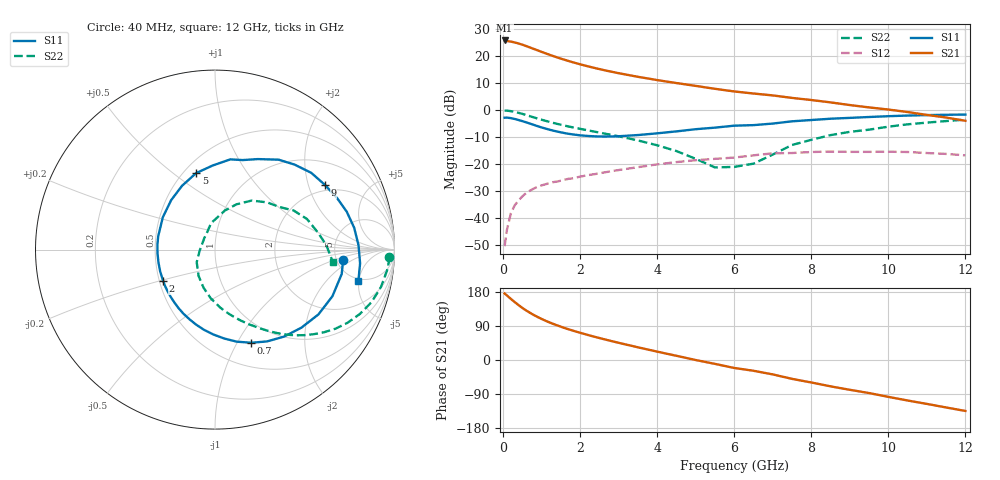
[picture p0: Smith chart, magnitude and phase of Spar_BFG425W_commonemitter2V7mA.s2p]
! Filename: 27bfg425.001
! BFG425W Field C1
! V1=8.380E-001V,V2=2.000E+000V, I1=9.357E-005A, I2=6.990E-003A
# GHz  S  MA  R 50
!  S11  S21  S12  S22
!Freq(GHz)  Mag  Ang  Mag  Ang  Mag  Ang  Mag  Ang
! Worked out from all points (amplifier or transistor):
!   44 points, 40 MHz to 12 GHz, reference 50 ohm
!   highest |S21| = 25.7 dB at 40 MHz (marker M1)
!   |S21| within 3 dB of that: start of sweep to 772.9 MHz
!   unconditionally stable (mu >= 1): 2.179 GHz to end of sweep
!   at 700 MHz: K = 0.42, MSG = 26.5 dB, |S12| = -29.9 dB
!   at 2.4 GHz: K = 1.06, MAG = 18.1 dB, |S12| = -23.7 dB
!   at 12 GHz: K = 1.43, MAG = 2.5 dB, |S12| = -16.8 dB
!   S11 on the Smith chart (normalised r, x): 40 MHz: 5.73, -1.33; 700 MHz: 0.76, -1.15; 2 GHz: 0.52, -0.21; 5 GHz: 0.58, +0.61; 9 GHz: 1.77, +2.58; 12 GHz: 4.61, -4.92
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0.04  0.716 -4.5  19.28 175.5  0.003 83.5  0.973 -2.4
0.2  0.704 -21.7  18.38 161.3  0.012 77.7  0.948 -12.7
0.3  0.68 -32.1  17.73 153.1  0.017 72.7  0.92 -18.6
0.4  0.649 -42.0  16.95 145.1  0.021 67.8  0.883 -24.0
0.5  0.619 -51.5  16.11 137.4  0.025 63.5  0.844 -28.8
0.6  0.588 -60.5  15.18 130.6  0.029 59.6  0.804 -33.2
0.7  0.557 -68.7  14.27 124.5  0.032 56.2  0.763 -37.1
0.9  0.498 -84.1  12.62 113.3  0.038 51.1  0.69 -43.7
1.2  0.431 -104.2  10.51 99.4  0.044 45.6  0.601 -51.5
1.4  0.398 -116.2  9.383 91.5  0.047 43.1  0.552 -55.8
1.6  0.371 -127.7  8.446 84.4  0.051 41.1  0.511 -59.6
2  0.338 -148.5  6.979 71.8  0.058 37.7  0.446 -66.9
2.2  0.329 -158.1  6.407 66.1  0.062 36.1  0.418 -70.4
3  0.325 166.9  4.775 45.4  0.077 29.2  0.324 -84.9
3.5  0.342 148.2  4.094 33.5  0.087 24.0  0.272 -95.1
4.5  0.4 117.4  3.138 11.1  0.108 11.6  0.173 -121.9
5  0.439 103.8  2.78 -0.1  0.117 3.9  0.124 -145.2
6.5  0.522 72.8  2.009 -28.4  0.144 -13.1  0.101 117.5
8.5  0.686 38.6  1.376 -69.5  0.169 -49.0  0.341 53.2
9  0.711 30.4  1.228 -78.7  0.167 -57.2  0.392 42.2
10.5  0.785 8.9  0.912 -106.9  0.166 -83.7  0.54 18.4
12  0.818 -12.5  0.628 -134.5  0.144 -113.6  0.66 -6.0
